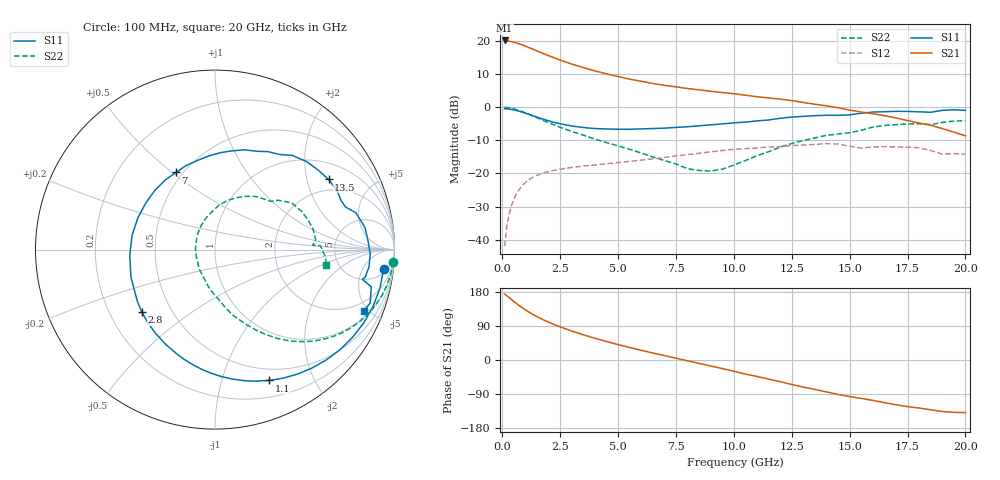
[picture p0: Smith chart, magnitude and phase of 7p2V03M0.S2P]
! Infineon Technologies  Discrete & RF Semiconductors
! bfp620
! VCE =  2.0 V,  IC =  3.0 mA
! Common Emitter S-Parameters:  Sep 2002
# GHz  S  MA  R  50
!  f  S11  S21  S12  S22
! GHz  MAG  ANG  MAG  ANG  MAG  ANG  MAG  ANG
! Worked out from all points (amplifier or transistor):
!   59 points, 100 MHz to 20 GHz, reference 50 ohm
!   highest |S21| = 20.1 dB at 100 MHz (marker M1)
!   |S21| within 3 dB of that: start of sweep to 1.441 GHz
!   unconditionally stable (mu >= 1): 5.348 GHz to 12.32 GHz; 14.33 GHz to 15.58 GHz; 17.37 GHz to end of sweep
!   at 1 GHz: K = 0.21, MSG = 20.6 dB, |S12| = -22.7 dB
!   at 5.5 GHz: K = 1.02, MAG = 11.6 dB, |S12| = -16.4 dB
!   at 20 GHz: K = 1.34, MAG = -0.7 dB, |S12| = -14.2 dB
!   S11 on the Smith chart (normalised r, x): 100 MHz: 7, -14; 1.1 GHz: 0.37, -1.43; 2.8 GHz: 0.34, -0.33; 7 GHz: 0.46, +0.52; 13.5 GHz: 1.55, +2.72; 20 GHz: 1.36, -4.67
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0.1  0.9457 -6.7  10.15 174.3  0.008 85.8  0.9944 -4.0
0.3  0.9359 -19.7  9.885 164.3  0.0249 78.7  0.9777 -11.9
0.5  0.9091 -32.5  9.538 154.3  0.0409 71.9  0.9445 -19.5
0.6  0.8919 -38.8  9.332 149.6  0.0483 68.5  0.9234 -23.1
0.8  0.8529 -50.7  8.861 140.6  0.0616 61.9  0.8751 -29.8
1.1  0.789 -67.5  8.068 128.4  0.078 53.0  0.795 -38.5
1.5  0.7067 -87.5  7.044 114.4  0.0938 43.4  0.6913 -47.8
1.9  0.637 -105.2  6.177 102.6  0.1045 36.2  0.6029 -55.0
2.4  0.5731 -125.0  5.284 89.7  0.1143 29.4  0.5131 -62.2
2.8  0.5365 -139.5  4.728 80.9  0.1202 25.1  0.4543 -67.1
3.5  0.493 -161.8  3.955 66.5  0.1294 19.0  0.3791 -74.7
4  0.4761 -176.1  3.524 57.4  0.1345 15.4  0.3293 -79.7
5  0.4647 157.9  2.895 40.6  0.146 9.9  0.2609 -88.8
6  0.4699 135.9  2.456 25.6  0.1589 4.6  0.2034 -101.5
7  0.4819 116.9  2.137 11.7  0.1743 -0.5  0.1568 -116.9
9  0.5415 86.6  1.739 -15.8  0.2119 -14.1  0.1089 175.6
10.5  0.5952 67.0  1.514 -37.2  0.2371 -27.9  0.1568 118.9
12  0.6792 50.6  1.323 -57.2  0.2545 -40.3  0.2492 84.8
13.5  0.7439 31.7  1.106 -77.6  0.2744 -55.0  0.3439 59.7
15  0.7647 18.1  0.904 -96.6  0.2576 -74.4  0.4121 40.7
17  0.8653 -1.7  0.689 -118.1  0.2511 -85.9  0.5453 17.2
20  0.8955 -22.4  0.37 -138.9  0.1956 -103.7  0.6264 -8.0
